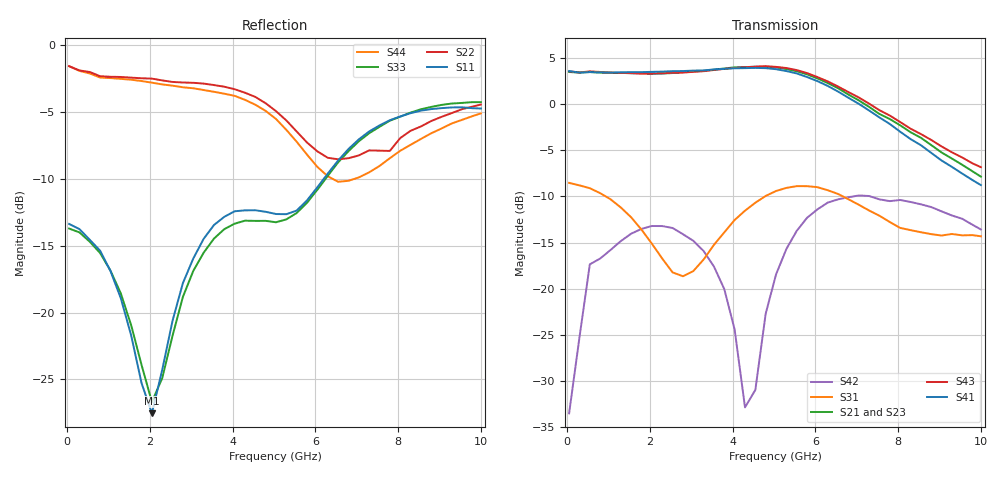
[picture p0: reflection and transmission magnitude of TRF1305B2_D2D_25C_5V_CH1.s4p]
!Created with skrf (http://scikit-rf.org).
! PORT[1] = INP
! PORT[2] = OUTM
! PORT[3] = INM
! PORT[4] = OUTP
# Hz S MA R 50.0
!freq magS11 angS11 magS12 angS12 magS13 angS13
! magS14 angS14
! magS21 angS21 magS22 angS22 magS23 angS23
! magS24 angS24
! magS31 angS31 magS32 angS32 magS33 angS33
! magS34 angS34
! magS41 angS41 magS42 angS42 magS43 angS43
! magS44 angS44
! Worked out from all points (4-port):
!   41 points, 50 MHz to 10 GHz, reference 50 ohm
!   strongest paths, dB at 50 MHz, 2.55 GHz, 5.05 GHz, 7.55 GHz, 10 GHz:
!     S41: 3.6, 3.6, 3.8, -1.4, -8.8
!     S43: 3.6, 3.4, 4.1, -0.6, -6.8
!     S21: 3.5, 3.4, 4.0, -1.1, -7.9
!     S23: 3.5, 3.4, 3.8, -1.5, -7.8
!     S31: -8.5, -18.2, -9.4, -12.1, -14.3
!     S42: -33.5, -13.4, -18.5, -10.3, -13.6
!   lowest |S11| = -27.5 dB at 2.05 GHz (marker M1), VSWR 1.09, Z = 54.2 + j1.15 ohm
!   |S11| at or under -10 dB: start of sweep to 6.205 GHz
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5e7  0.2144 -2.5  0.004354 4.4  0.3712 -2.2  0.001596 106.1
     1.496 177.4  0.8334 177.6  1.492 -2.2  0.01893 111.9
     0.3745 -2.4  0.003433 113.5  0.2061 -1.4  0.001737 31.3
     1.514 -2.5  0.02107 116.2  1.508 177.5  0.8332 177.2
2.05e9  0.04202 14.6  0.04209 -23.3  0.175 -101.0  0.03159 -43.4
        1.465 76.8  0.7488 108.0  1.471 -100.8  0.2179 1.5
        0.1752 -104.6  0.02922 -48.9  0.04634 -1.0  0.04557 -23.5
        1.498 -100.9  0.2186 3.0  1.468 76.4  0.7231 109.7
3.55e9  0.2124 35.5  0.05361 -74.0  0.1686 115.1  0.0376 -123.5
        1.542 0.8  0.7085 66.6  1.526 -177.0  0.1327 -53.3
        0.1728 110.6  0.03426 -125.2  0.189 33.8  0.05803 -76.3
        1.544 -177.7  0.1317 -51.5  1.534 0.6  0.6685 68.0
5.05e9  0.2335 10.8  0.06663 -123.2  0.3431 45.4  0.03359 151.0
        1.584 -84.9  0.566 29.6  1.545 97.2  0.1235 89.4
        0.3384 42.5  0.03038 147.2  0.2175 12.8  0.07115 -123.9
        1.549 96.7  0.1193 83.1  1.595 -83.7  0.5289 28.7
6.55e9  0.3699 9.8  0.07565 177.4  0.3326 -5.1  0.01688 60.1
        1.221 -174.6  0.374 25.9  1.17 6.7  0.3129 25.2
        0.3261 -6.5  0.01533 56.1  0.3642 8.5  0.08029 178.4
        1.171 5.2  0.3049 22.0  1.247 -173.0  0.3082 24.7
8.3e9  0.5561 -34.9  0.07421 115.2  0.2126 -24.5  0.003046 -134.6
       0.7053 97.1  0.4778 27.4  0.6805 -83.7  0.3041 -20.2
       0.2076 -25.7  0.001709 -95.4  0.5588 -36.7  0.07872 115.1
       0.6474 -87.5  0.2951 -22.1  0.7372 99.2  0.4234 28.6
1e10  0.579 -81.5  0.07719 56.8  0.201 -37.0  0.01311 110.1
      0.4049 27.3  0.5991 4.5  0.4069 -160.8  0.2223 -53.3
      0.1922 -37.3  0.01044 100.5  0.6115 -86.2  0.07868 59.5
      0.3643 -162.2  0.2094 -53.2  0.4557 28.9  0.555 5.9
